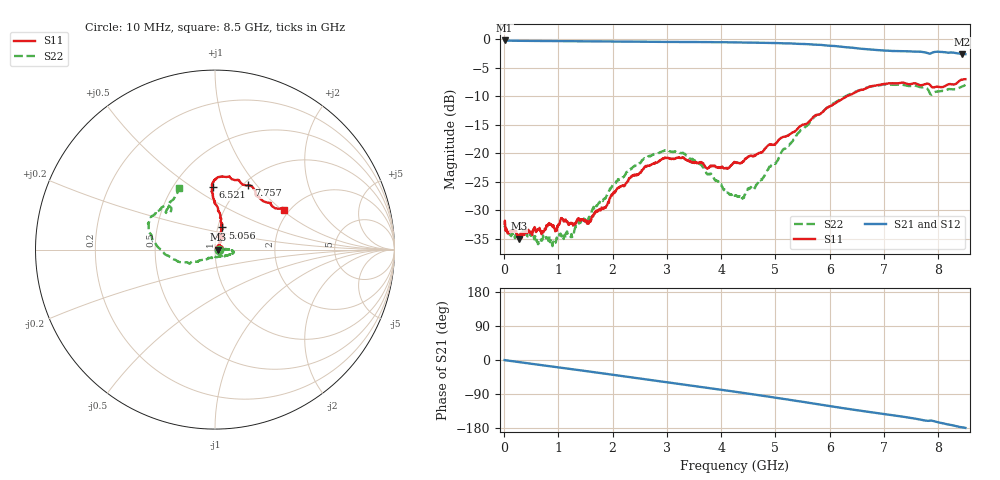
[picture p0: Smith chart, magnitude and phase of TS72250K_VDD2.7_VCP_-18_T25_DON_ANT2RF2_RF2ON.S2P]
!Agilent Technologies,E5071C,MY46417908,A.11.23
!Date: Thu Oct 03 13:33:48 2019
!Data & Calibration Information:
!Freq	S11:SOLT2(ON)	S21:SOLT2(ON)	S12:SOLT2(ON)	S22:SOLT2(ON)
!PortZ  Port1:50+j0  Port2:50+j0
!Above PortZ is port z conversion or system Z0 setting when saving the data.
!When reading, reference impedance value at option line is always used.
# Hz S dB R 50
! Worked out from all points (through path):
!   1601 points, 10 MHz to 8.5 GHz, reference 50 ohm
!   highest |S21| = -0.23 dB at 10 MHz (marker M1); lowest = -2.6 dB at 8.442 GHz (marker M2)
!   group delay of S21, straight-line fit = 57.6 ps
!   lowest |S11| = -35.0 dB at 270 MHz (marker M3), VSWR 1.04, Z = 51.8 + j0.0547 ohm
!   |S11| at or under -10 dB: start of sweep to 6.318 GHz
!   |S22| runs from -36.3 to -7.9 dB; largest |S21 - S12| = 0.0048
!   S11 on the Smith chart (normalised r, x): 10 MHz: 1.05, +0.01; 5.056 GHz: 1.05, +0.26; 6.521 GHz: 0.76, +0.61; 7.757 GHz: 1.06, +0.90; 8.5 GHz: 1.88, +1.05
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1e7  -32.33 10.1  -0.23 -0.3  -0.24 -0.2  -33.01 -9.1
2.700062e8  -34.96 1.7  -0.30 -5.4  -0.31 -5.3  -34.66 4.0
9.120625e8  -32.78 12.3  -0.34 -17.8  -0.34 -17.8  -35.56 34.0
1.081862e9  -31.54 18.1  -0.35 -21.0  -0.35 -21.0  -34.73 31.9
1.246356e9  -32.22 21.3  -0.35 -24.2  -0.36 -24.2  -34.64 22.4
1.426769e9  -31.74 36.5  -0.37 -27.7  -0.37 -27.7  -31.71 17.3
1.570038e9  -31.95 41.9  -0.37 -30.5  -0.38 -30.5  -31.43 8.1
2.291688e9  -24.77 59.7  -0.43 -44.5  -0.43 -44.5  -23.00 -0.6
2.843538e9  -21.46 60.9  -0.48 -55.3  -0.48 -55.4  -19.98 -6.4
3.331712e9  -21.05 60.8  -0.50 -65.0  -0.50 -65.1  -20.12 -12.3
3.7456e9  -22.63 68.1  -0.53 -73.3  -0.53 -73.3  -23.69 -29.3
4.255e9  -21.58 74.1  -0.58 -83.7  -0.59 -83.7  -27.40 -74.4
4.387656e9  -21.57 74.0  -0.58 -86.5  -0.59 -86.5  -27.95 -91.5
4.605212e9  -20.45 71.5  -0.62 -90.9  -0.62 -91.0  -26.27 -113.6
5.056244e9  -17.71 71.4  -0.70 -100.7  -0.68 -100.7  -20.97 -140.1
5.671769e9  -13.94 82.1  -0.94 -114.2  -0.94 -114.2  -14.15 -158.5
6.520769e9  -9.10 92.1  -1.63 -132.9  -1.66 -132.9  -9.04 170.7
7.088538e9  -7.77 84.8  -2.02 -144.3  -2.04 -144.5  -7.98 157.5
7.757125e9  -7.88 62.7  -2.32 -159.7  -2.29 -159.6  -8.46 141.1
7.884475e9  -8.42 53.3  -2.39 -160.2  -2.39 -160.0  -9.70 141.4
8.441631e9  -7.10 31.6  -2.63 -177.6  -2.66 -177.8  -8.29 121.7
8.5e9  -7.02 30.1  -2.63 -179.2  -2.66 -179.4  -8.01 120.6
